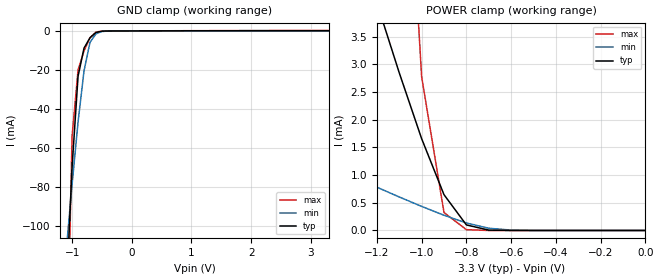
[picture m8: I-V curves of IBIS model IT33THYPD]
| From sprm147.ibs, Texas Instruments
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[Model]   IT33THYPD
Model_type   Input
Polarity   Non-Inverting
| signals   A, Y
Vinl = 0.8V
Vinh = 2.0V
|   typ   min   max
C_comp   0.89711294p   0.86828627p   0.92483787p
|   typ   min   max
[Temperature Range]   25   -40   125
|   typ   min   max
[Voltage Range]   3.30V   3.00V   3.60V
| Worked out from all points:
|   GND clamp passes 1 mA (typ) near -0.61 V on its own axis
|   POWER clamp passes 1 mA (typ) near -0.93 V on its own axis
[GND_clamp]
|   Voltage   I(typ)   I(min)   I(max)
-3.3V     -1.935A    -960.6mA   -4.953A
-1.1V     -136.6mA   -113.2mA   -192.9mA
-1V       -69.73mA   -78.71mA   -53.93mA
-900mV    -23.26mA   -46.75mA   -20.01mA
-800mV    -8.808mA   -20.45mA   -10.25mA
-700mV    -3.5mA     -5.867mA   -3.497mA
-600mV    -809.8uA   -1.501mA   -569.6uA
-500mV    -122.5uA   -299.8uA   -100.3uA
-400mV    -40.39uA   -55.28uA   -57.69uA
3.3V      101.5uA    52.27uA    182uA
[POWER_clamp]
|   Voltage   I(typ)   I(min)   I(max)
-3.3V     33.03mA    4.773mA    224.5mA
-2.7V     24.64mA    3.607mA    164.7mA
-1.8V     12.17mA    1.89mA     75.57mA
-1.2V     4.113mA    781.6uA    18.29mA
-1.1V     2.848mA    605.4uA    9.702mA
-1V       1.658mA    435uA      2.778mA
-900mV    646uA      274.8uA    323.3uA
-800mV    100.4uA    135.2uA    14.29uA
-700mV    6.235uA    40.32uA    116.8nA
-600mV    176.8nA    6.906uA    888.2pA
-500mV    5.063nA    714.3nA    88.82pA
0V        1pA        1pA        1pA
